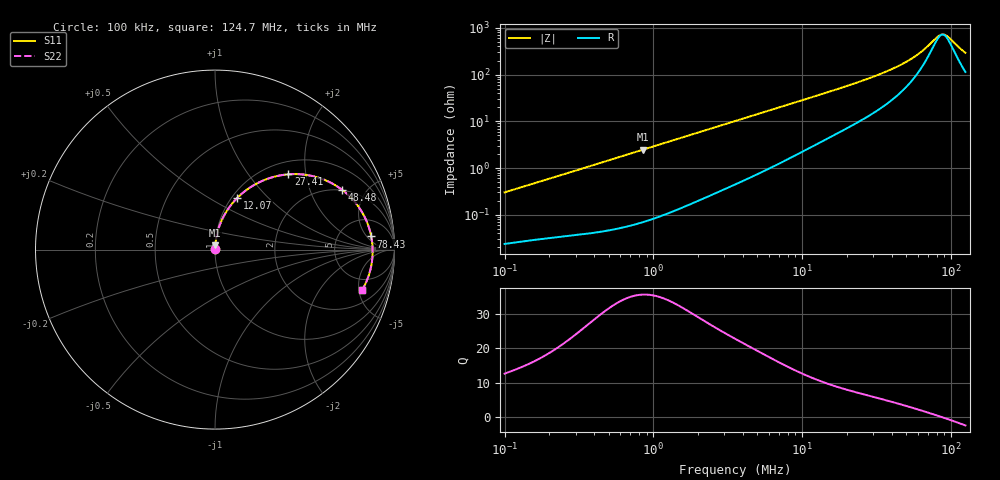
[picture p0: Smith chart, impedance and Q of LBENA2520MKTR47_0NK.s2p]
! LBENA2520MKTR47_0NK  S-PARAMETER MODEL  ( General Type )
! Model Generated by TAIYO YUDEN Corporation (http://www.ty-top.com)
! Version 1.0
! TAIYO YUDEN Control No. 211116
! Copyright(c) 2021 TAIYO YUDEN CO.,LTD. All Rights Reserved.
! Product Description (link to TY-COMPAS)
! https://ds.yuden.co.jp/TYCOMPAS/or/detail?pn=LBENA2520MKTR47M0NK&u=M
! Products Name : Inductors
! Characteristics :
!  Inductance : 0.47 uH , SRF(min) : -Hz , DC Resistance(max) : 0.02 Ohm
!  Rated Current : Saturation :5900 mA , Temp Rise : 5000 mA
!  Case Size : 2.5 x 2.0 / 0.098 x 0.079 [mm/inch] , Thickness : 1.2 / 0.047 [mm/inch]
!  (Conditions: Temperature = 25 degC , DC Bias Current/Voltage = 0A / 0V)
! External Node Assignments :
!  1  o---GGG---o  2
! GND o---------o GND
! Frequency Range : 0.1MHz  -  124.6553MHz  [ 402 STEP ]
# MHz S RI R 50
! Freq[MHz].  S11 Real  S11 Imag  S21 Real  S21 Imag  S12 Real  S12 Imag  S22 Real  S22 Imag
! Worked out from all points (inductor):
!   401 points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, 100 kHz to 124.7 MHz, reference 50 ohm
!   read as one part in series: L = 475 nH near 103.6 kHz
!   highest Q = 35.6 at 848.6 kHz (marker M1), where L = 463 nH
!   self-resonance near 87.55 MHz
!   S11 on the Smith chart (normalised r, x): 100 kHz: 1.00, +0.01; 12.07 MHz: 1.06, +0.68; 27.41 MHz: 1.25, +1.60; 48.48 MHz: 1.99, +3.41; 78.43 MHz: 11, +7; 124.7 MHz: 3.28, -5.37
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0.1  0.000247 0.00301  0.9998 -0.00301  0.9998 -0.00301  0.000247 0.00301
0.330013  0.000473 0.00966  0.9995 -0.00966  0.9995 -0.00966  0.000473 0.00966
0.84862  0.0013 0.0246  0.9987 -0.0246  0.9987 -0.0246  0.0013 0.0246
1.089088  0.0019 0.0315  0.9981 -0.0315  0.9981 -0.0315  0.0019 0.0315
3.530656  0.0144 0.099  0.9856 -0.099  0.9856 -0.099  0.0144 0.099
6.949409  0.0481 0.1849  0.9519 -0.1849  0.9519 -0.1849  0.0481 0.1849
11.65164  0.1176 0.2814  0.8824 -0.2814  0.8824 -0.2814  0.1176 0.2814
12.0744  0.1248 0.2887  0.8752 -0.2887  0.8752 -0.2887  0.1248 0.2887
18.19151  0.2365 0.3702  0.7635 -0.3702  0.7635 -0.3702  0.2365 0.3702
27.40768  0.4094 0.4195  0.5906 -0.4195  0.5906 -0.4195  0.4094 0.4195
38.45196  0.5882 0.3969  0.4118 -0.3969  0.4118 -0.3969  0.5882 0.3969
48.47626  0.7097 0.3319  0.2903 -0.3319  0.2903 -0.3319  0.7097 0.3319
54.91665  0.7673 0.279  0.2327 -0.279  0.2327 -0.279  0.7673 0.279
62.21269  0.8154 0.2149  0.1846 -0.2149  0.1846 -0.2149  0.8154 0.2149
69.23323  0.8469 0.1525  0.1531 -0.1525  0.1531 -0.1525  0.8469 0.1525
78.43133  0.8705 0.0732  0.1295 -0.0732  0.1295 -0.0732  0.8705 0.0732
85.74049  0.8778 0.014  0.1222 -0.014  0.1222 -0.014  0.8778 0.014
88.85144  0.8784 -0.00998  0.1216 0.00998  0.1216 0.00998  0.8784 -0.00998
92.07528  0.8777 -0.034  0.1223 0.034  0.1223 0.034  0.8777 -0.034
97.13167  0.874 -0.0698  0.126 0.0698  0.126 0.0698  0.874 -0.0698
116.079  0.8406 -0.185  0.1594 0.185  0.1594 0.185  0.8406 -0.185
124.6553  0.8186 -0.2276  0.1814 0.2276  0.1814 0.2276  0.8186 -0.2276
